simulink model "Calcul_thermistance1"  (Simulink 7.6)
settings: Solver=ode15s  StartTime=0.0  StopTime=10.0  RelTol=1e-3
InitFcn:
  | R1=1e3;
  | R2=2*R1;
  | 
  | Vcc=12;
libraries: fl_lib x13, nesl_utility x2, elec_lib x1

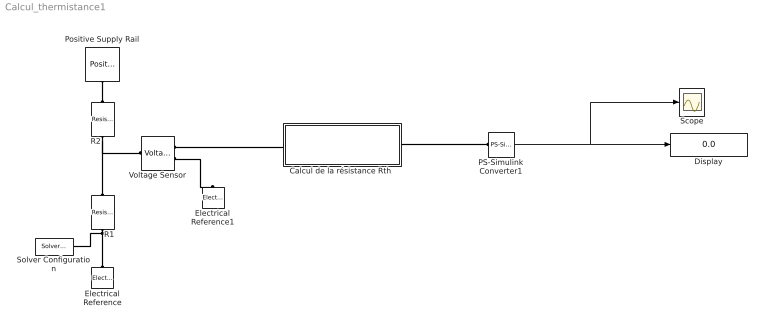
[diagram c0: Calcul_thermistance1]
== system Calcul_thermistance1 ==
  "Calcul de la résistance Rth " : Subsystem
  Display : Display
  Electrical Reference : fl_lib/Electrical/Electrical Elements/Electrical Reference  DialogController=NetworkEngine.DynNeDlgSource  SystemSampleTime=-1  i_Log=off  LocalVarNames=|i  LocalVarDescs=|i  LocalVarLogging=[]
  Electrical Reference1 : fl_lib/Electrical/Electrical Elements/Electrical Reference  DialogController=NetworkEngine.DynNeDlgSource  SystemSampleTime=-1  i_Log=off  LocalVarNames=|i  LocalVarDescs=|i  LocalVarLogging=[]
  PS-Simulink Converter1 : nesl_utility/PS-Simulink Converter  DialogController=NetworkEngine.DynNeUtilDlgSource  SystemSampleTime=-1  PhysicalDomain=network_engine_domain  LeftPortType=input  RightPortType=output  SubClassName=ps_output  Unit=V  AffineConversion=off
  Positive Supply Rail : elec_lib/Sources/Positive Supply Rail  DialogController=NetworkEngine.DynNeDlgSource  SystemSampleTime=-1  v0=Vcc V  current_Log=off  voltage_Log=off  power_Log=off  LocalVarNames=|current|voltage|power  LocalVarDescs=|Current (A)|Voltage (V)|Power (W)  LocalVarLogging=[0 0 0]
  R1 : fl_lib/Electrical/Electrical Elements/Resistor  DialogController=NetworkEngine.DynNeDlgSource  SystemSampleTime=-1  R=R1 kOhm  i_Log=off  v_Log=off  LocalVarNames=|current|voltage|power  LocalVarDescs=|Resistor current (A)|Voltage across resistor (V)|Power (W)  LocalVarLogging=[0 0 0]
  R2 : fl_lib/Electrical/Electrical Elements/Resistor  DialogController=NetworkEngine.DynNeDlgSource  SystemSampleTime=-1  R=R2 kOhm  i_Log=off  v_Log=off  LocalVarNames=|current|voltage|power  LocalVarDescs=|Resistor current (A)|Voltage across resistor (V)|Power (W)  LocalVarLogging=[0 0 0]
  Scope : Scope
  Solver Configuration : nesl_utility/Solver Configuration  DialogController=NetworkEngine.DynNeUtilDlgSource  SystemSampleTime=-1  PhysicalDomain=network_engine_domain  LeftPortType=input  RightPortType=generic  SubClassName=solver  Accelerate=off  Profile=off  ResidualTolerance=1e-9  MaxNonlinIter=12  MaxModeIter=2  DoFixedCost=off  UseLocalSampling=off  DoDC=off  LinearAlgebra=Sparse  LocalSolverSampleTime=.001  LocalSolverChoice=NE_BACKWARD_EULER_ADVANCER  UseLocalSolver=off
  Voltage Sensor : fl_lib/Electrical/Electrical Sensors/Voltage Sensor  DialogController=NetworkEngine.DynNeDlgSource  SystemSampleTime=-1  i1_Log=off  v1_Log=off  LocalVarNames=|i1|v1  LocalVarDescs=|i1|v1  LocalVarLogging=[]
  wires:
  PS-Simulink Converter1/1 -> Display/1, Scope/1
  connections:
  Voltage Sensor/RConn2 -- Electrical Reference1/LConn1
  Positive Supply Rail/RConn1 -- R2/RConn1
  R2/LConn1 -- R1/RConn1 -- Voltage Sensor/LConn1
  R1/LConn1 -- Electrical Reference/LConn1 -- Solver Configuration/RConn1
  PS-Simulink Converter1/LConn1 -- "Calcul de la résistance Rth "/RConn1
  "Calcul de la résistance Rth "/LConn1 -- Voltage Sensor/RConn1

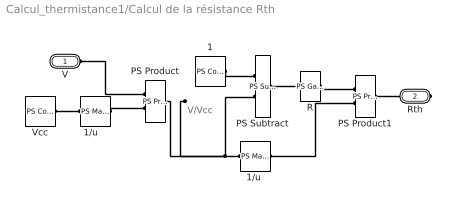
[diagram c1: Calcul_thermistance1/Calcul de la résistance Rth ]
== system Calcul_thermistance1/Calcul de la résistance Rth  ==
  note: V/Vcc
  1 : fl_lib/Physical Signals/Sources/PS Constant  DialogController=NetworkEngine.DynNeDlgSource  SystemSampleTime=-1  constant=1  LocalVarLogging=[]
  "1/u " : fl_lib/Physical Signals/Functions/PS Math Function  DialogController=NetworkEngine.DynNeDlgSource  SystemSampleTime=-1  fcn_choice=9  LocalVarLogging=[]
  "1/u   " : fl_lib/Physical Signals/Functions/PS Math Function  DialogController=NetworkEngine.DynNeDlgSource  SystemSampleTime=-1  fcn_choice=9  LocalVarLogging=[]
  PS Product : fl_lib/Physical Signals/Functions/PS Product  DialogController=NetworkEngine.DynNeDlgSource  SystemSampleTime=-1  LocalVarLogging=[]
  PS Product1 : fl_lib/Physical Signals/Functions/PS Product  DialogController=NetworkEngine.DynNeDlgSource  SystemSampleTime=-1  LocalVarLogging=[]
  PS Subtract : fl_lib/Physical Signals/Functions/PS Subtract  DialogController=NetworkEngine.DynNeDlgSource  SystemSampleTime=-1  LocalVarLogging=[]
  R : fl_lib/Physical Signals/Functions/PS Gain  DialogController=NetworkEngine.DynNeDlgSource  SystemSampleTime=-1  gain=R1  LocalVarLogging=[]
  Vcc : fl_lib/Physical Signals/Sources/PS Constant  DialogController=NetworkEngine.DynNeDlgSource  SystemSampleTime=-1  constant=Vcc  LocalVarLogging=[]
  V : PMIOPort  Port=1  Side=Left
  Rth : PMIOPort  Port=2  Side=Right
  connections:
  1/RConn1 -- PS Subtract/LConn1
  "1/u "/LConn1 -- PS Product/RConn1 -- PS Subtract/LConn2
  "1/u "/RConn1 -- PS Product1/LConn2
  Vcc/RConn1 -- "1/u   "/LConn1
  "1/u   "/RConn1 -- PS Product/LConn2
  R/RConn1 -- PS Product1/LConn1
  PS Subtract/RConn1 -- R/LConn1
  V/RConn1 -- PS Product/LConn1
  Rth/RConn1 -- PS Product1/RConn1
